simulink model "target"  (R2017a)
settings: Solver=FixedStepDiscrete  StartTime=0.0  StopTime=inf  FixedStep=0.01  RelTol=1e-3  EnableMultiTasking=on
libraries: c280xlib x2

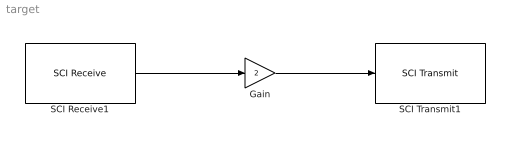
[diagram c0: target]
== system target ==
  Gain : Gain  Gain=2  OutDataTypeStr=single
  SCI Receive1 : c280xlib/SCI Receive  sciModule=B  dataHead='S'  dataTail='E'  dataType=single  dataDim=1  initValue=0  errOption=Output the last received value  errValue=0  sampleTime=0.1  outputStatus=off  postInterrupt=off  numFifo=1
  SCI Transmit1 : c280xlib/SCI Transmit  sciModule=B  dataHead='S'  dataTail='E'  postInterrupt=off  numFifo=1
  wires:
  Gain/1 -> SCI Transmit1/1
  SCI Receive1/1 -> Gain/1
